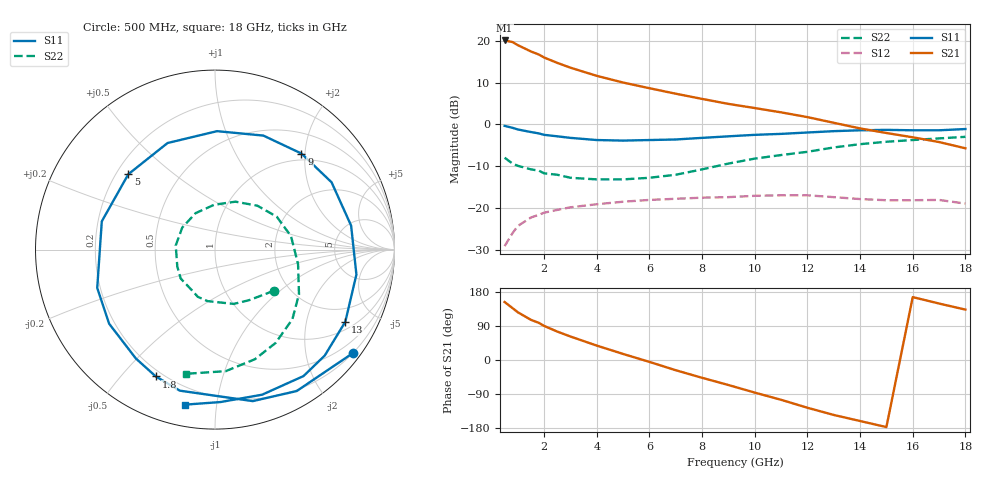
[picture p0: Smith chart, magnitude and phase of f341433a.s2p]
!ATF-34143
!S-PARAMETERS at Vds=3V  Id=20mA.  LAST UPDATED 01-29-99
# ghz s ma r 50
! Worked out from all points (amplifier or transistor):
!   23 points, 500 MHz to 18 GHz, reference 50 ohm
!   highest |S21| = 20.1 dB at 500 MHz (marker M1)
!   |S21| within 3 dB of that: start of sweep to 1.651 GHz
!   unconditionally stable (mu >= 1): 6.267 GHz to end of sweep
!   at 1.5 GHz: K = 0.34, MSG = 19.9 dB, |S12| = -22.3 dB
!   at 7 GHz: K = 1.07, MAG = 10.9 dB, |S12| = -17.8 dB
!   at 18 GHz: K = 1.48, MAG = 2.5 dB, |S12| = -18.9 dB
!   lowest NFmin = 0.10 dB at 500 MHz
!   S11 on the Smith chart (normalised r, x): 500 MHz: 0.20, -2.98; 1.8 GHz: 0.17, -0.62; 5 GHz: 0.25, +0.35; 9 GHz: 0.87, +1.93; 13 GHz: 1.31, -3.40; 18 GHz: 0.11, -0.82
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0.5  0.96 -37.0  10.08 153.0  0.035 68.0  0.4 -35.0
0.8  0.91 -60.0  9.642 137.0  0.05 56.0  0.34 -56.0
1  0.87 -76.0  8.867 126.0  0.061 48.0  0.32 -71.0
1.5  0.81 -104.0  7.443 106.0  0.077 34.0  0.29 -98.0
1.8  0.78 -115.0  6.843 98.0  0.083 28.0  0.28 -110.0
2  0.75 -126.0  6.306 90.0  0.088 23.0  0.26 -120.0
2.5  0.72 -145.0  5.438 75.0  0.095 15.0  0.25 -140.0
3  0.69 -162.0  4.762 62.0  0.102 7.0  0.23 -156.0
4  0.65 166.0  3.806 38.0  0.111 -8.0  0.22 174.0
5  0.64 139.0  3.165 16.0  0.119 -21.0  0.22 146.0
6  0.65 114.0  2.706 -5.0  0.125 -35.0  0.23 118.0
7  0.66 89.0  2.326 -27.0  0.129 -49.0  0.25 91.0
8  0.69 67.0  2.017 -47.0  0.133 -62.0  0.29 67.0
9  0.72 48.0  1.758 -66.0  0.135 -75.0  0.34 46.0
10  0.75 30.0  1.568 -86.0  0.14 -88.0  0.39 28.0
11  0.77 10.0  1.393 -105.0  0.142 -103.0  0.43 10.0
12  0.8 -10.0  1.222 -126.0  0.142 -118.0  0.47 -10.0
13  0.83 -29.0  1.045 -145.0  0.135 -133.0  0.53 -28.0
15  0.86 -55.0  0.789 -177.0  0.124 -156.0  0.62 -57.0
16  0.85 -72.0  0.701 166.0  0.124 -168.0  0.65 -70.0
17  0.85 -88.0  0.615 149.0  0.125 177.0  0.68 -85.0
18  0.88 -101.0  0.518 133.0  0.113 165.0  0.71 -103.0
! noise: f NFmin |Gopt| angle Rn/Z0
0.5  0.1  0.9  13  0.16
0.9  0.11  0.85  27  0.14
1.5  0.14  0.77  48  0.11
1.8  0.17  0.74  57  0.1
2.5  0.23  0.65  83  0.07
3  0.29  0.59  102  0.06
5  0.54  0.45  174  0.03
6  0.67  0.42  -151  0.05
8  0.92  0.45  -88  0.18
10  1.16  0.61  -43  0.46
